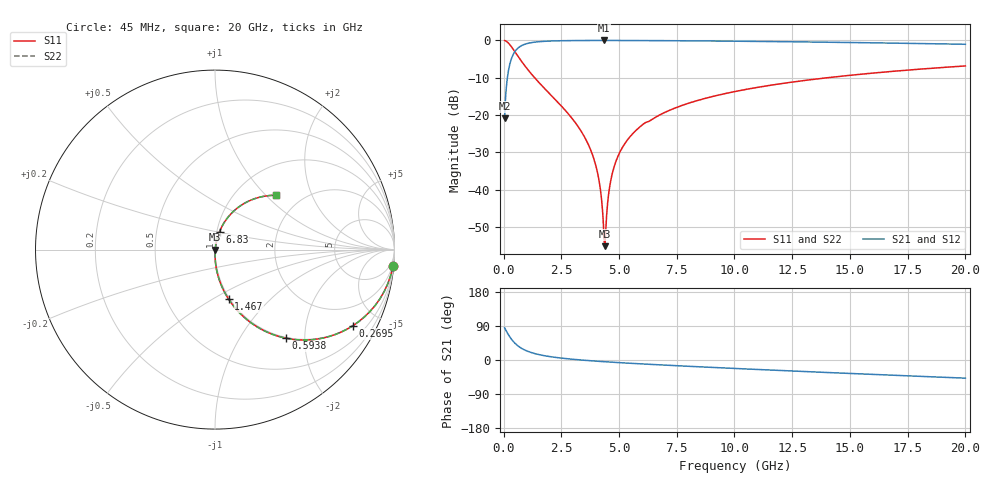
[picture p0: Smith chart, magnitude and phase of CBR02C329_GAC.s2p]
! S-parameter model data by Modelithics Inc.  support@modelithics.com 813-866-6335  Tampa FL USA
! S-Parameter data specifications:
! Substrate: 20-mil Rogers 4350B, substrate thickness, H=0.508mm, Dielectric constant, Er=3.75
! PCB Mounting Pad Footprint: Pad width, PadW=0.32mm , Pad length, PadL=0.37mm , Pad gap, PadG (edge-to-edge)=0.19mm , Reference planes=0.93mm apart
#  GHz  S  MA  R 50
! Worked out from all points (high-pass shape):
!   801 points, 45 MHz to 20 GHz, reference 50 ohm
!   highest |S21| = -0.02 dB at 4.335 GHz (marker M1); lowest = -20.9 dB at 45 MHz (marker M2)
!   |S21| within 3 dB of the highest: 489.1 MHz to end of sweep
!   lowest |S11| = -55.1 dB at 4.385 GHz (marker M3), VSWR 1.00, Z = 50.2 + j0.00712 ohm
!   |S11| at or under -10 dB: 1.345 GHz to 14.03 GHz (12.68 GHz wide, 165 % of centre)
!   |S22| runs from -55.1 to 0.0 dB; largest |S21 - S12| = 0
!   S11 on the Smith chart (normalised r, x): 45 MHz: 1, -22; 269.5 MHz: 0.98, -3.63; 593.8 MHz: 0.98, -1.62; 1.467 GHz: 0.99, -0.59; 6.83 GHz: 1.03, +0.21; 20 GHz: 1.50, +1.15
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0.045  0.9959 -5.2  0.09051 84.8  0.09051 84.8  0.9959 -5.2
0.194662  0.9303 -21.7  0.3664 68.3  0.3664 68.3  0.9303 -21.7
0.269494  0.8774 -28.9  0.4793 61.0  0.4793 61.0  0.8774 -28.9
0.593762  0.6331 -51.3  0.7733 38.7  0.7733 38.7  0.6331 -51.3
0.942975  0.4474 -64.3  0.8933 25.6  0.8933 25.6  0.4474 -64.3
1.466794  0.2869 -74.6  0.9567 15.1  0.9567 15.1  0.2869 -74.6
3.387462  0.05878 -88.6  0.9966 -0.2  0.9966 -0.2  0.05878 -88.6
4.011056  0.02009 -88.2  0.998 -3.0  0.998 -3.0  0.02009 -88.2
4.185663  0.01049 -84.4  0.9982 -3.8  0.9982 -3.8  0.01049 -84.4
4.335325  0.002946 -58.4  0.9982 -4.4  0.9982 -4.4  0.002946 -58.4
4.385212  0.00175 2.3  0.9982 -4.6  0.9982 -4.6  0.00175 2.3
4.460044  0.004409 61.8  0.9982 -4.9  0.9982 -4.9  0.004409 61.8
4.559819  0.00924 73.8  0.9981 -5.3  0.9981 -5.3  0.00924 73.8
4.659594  0.0141 77.1  0.998 -5.7  0.998 -5.7  0.0141 77.1
5.03375  0.0317 79.6  0.9976 -7.1  0.9976 -7.1  0.0317 79.6
5.732175  0.06212 78.6  0.9959 -9.5  0.9959 -9.5  0.06212 78.6
6.704981  0.09816 76.1  0.9928 -12.6  0.9928 -12.6  0.09816 76.1
6.8297  0.1028 75.8  0.9924 -13.0  0.9924 -13.0  0.1028 75.8
10.0225  0.2066 67.0  0.9759 -22.3  0.9759 -22.3  0.2066 67.0
13.36496  0.2991 58.2  0.9514 -31.3  0.9514 -31.3  0.2991 58.2
16.68248  0.381 49.8  0.9215 -39.8  0.9215 -39.8  0.381 49.8
20  0.4548 41.7  0.8873 -47.9  0.8873 -47.9  0.4548 41.7
